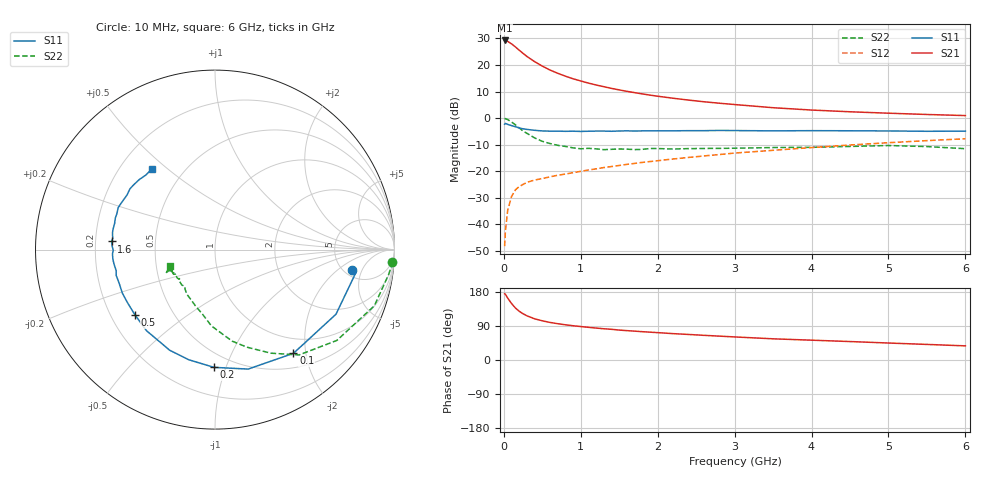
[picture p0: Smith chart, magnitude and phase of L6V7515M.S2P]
!  INFINEON TECHNOLOGIES Small Signal Semiconductors
! BFR380L3 , Si-NPN RF-Transistor in TSLP-3-1
!  Vce=0.75 V,  Ic=15 mA
! Common Emitter S-Parameters:  07. March 2005
#  GHz  S  MA  R  50
! f  S11  S21  S12  S22
! GHz  Mag  Ang  Mag  Ang  Mag  Ang  Mag  Ang
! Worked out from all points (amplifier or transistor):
!   36 points, 10 MHz to 6 GHz, reference 50 ohm
!   highest |S21| = 29.3 dB at 10 MHz (marker M1)
!   |S21| within 3 dB of that: start of sweep to 172.9 MHz
!   unconditionally stable (mu >= 1): 1.853 GHz to 5.429 GHz
!   at 250 MHz: K = 0.33, MSG = 24.7 dB, |S12| = -24.9 dB
!   at 1.4 GHz: K = 0.95, MSG = 14.7 dB, |S12| = -18.2 dB
!   at 6 GHz: K = 0.99, MSG = 4.4 dB, |S12| = -7.7 dB
!   S11 on the Smith chart (normalised r, x): 10 MHz: 5.89, -3.21; 100 MHz: 0.73, -1.78; 200 MHz: 0.39, -0.91; 500 MHz: 0.30, -0.33; 1.6 GHz: 0.27, +0.04; 6 GHz: 0.33, +0.45
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0.01  0.7695 -8.3  29.04 174.8  0.0039 77.8  0.9912 -4.0
0.02  0.7973 -8.8  28.79 173.5  0.0074 82.3  0.9777 -8.1
0.05  0.7642 -28.1  27.89 163.4  0.0185 78.2  0.9415 -19.4
0.1  0.7246 -52.9  25.06 149.1  0.0335 66.2  0.8468 -36.7
0.15  0.6908 -74.5  21.97 137.3  0.0447 57.4  0.7509 -51.4
0.2  0.6561 -90.5  19 128.6  0.0518 53.5  0.6561 -61.6
0.25  0.6307 -103.5  16.6 122.0  0.0567 49.0  0.5725 -71.8
0.3  0.615 -114.2  14.52 116.6  0.062 47.6  0.5188 -79.4
0.4  0.5914 -130.2  11.59 108.7  0.0685 45.2  0.4255 -92.7
0.5  0.5754 -140.9  9.556 103.4  0.0732 46.0  0.3668 -100.9
0.6  0.5702 -149.1  8.059 99.1  0.0787 46.4  0.3332 -108.8
0.8  0.5659 -160.7  6.182 92.9  0.0888 48.9  0.2939 -122.3
0.9  0.5689 -165.3  5.515 90.4  0.0942 49.9  0.2764 -127.1
1.1  0.5679 -171.5  4.576 86.2  0.106 52.6  0.2706 -133.3
1.3  0.5717 -177.7  3.913 82.4  0.1177 54.2  0.2556 -140.8
1.6  0.5779 175.5  3.201 77.5  0.1352 56.2  0.2613 -147.4
2.2  0.578 165.4  2.375 69.6  0.1705 58.4  0.2629 -150.7
2.8  0.5877 156.6  1.914 63.0  0.2068 59.6  0.2703 -155.8
3.5  0.577 148.1  1.574 55.9  0.2486 58.5  0.2801 -155.2
4.5  0.5793 141.5  1.32 48.7  0.3125 57.5  0.2937 -155.0
5.5  0.5667 133.0  1.174 41.1  0.3779 54.0  0.292 -155.9
6  0.5707 127.7  1.12 37.3  0.4102 52.0  0.2664 -160.0
